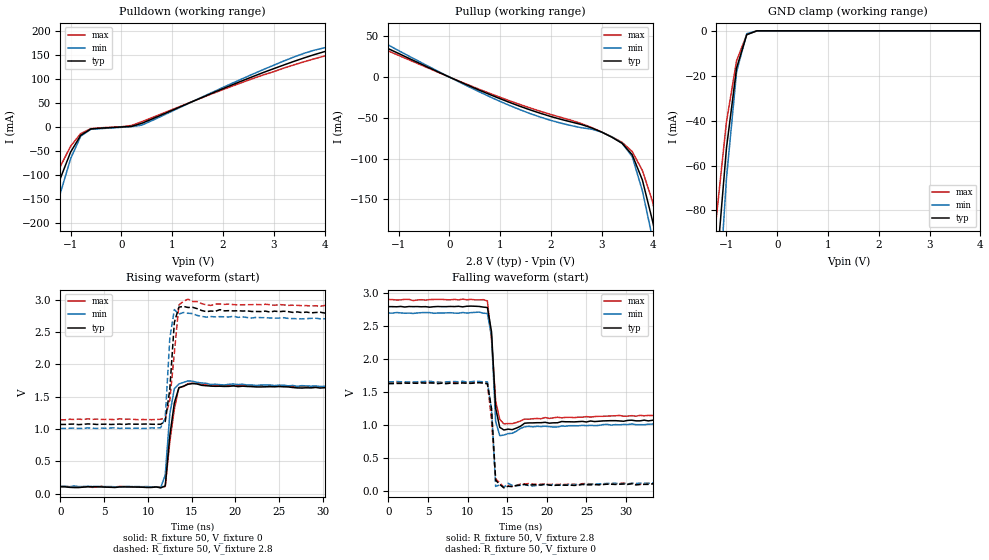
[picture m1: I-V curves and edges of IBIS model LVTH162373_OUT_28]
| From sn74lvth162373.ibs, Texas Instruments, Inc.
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|  Model LVTH162373 OUTPUT_28
[Model]   LVTH162373_OUT_28
Model_type  3-state
Polarity   Non-Inverting
Enable   Active-Low
Vmeas = 1.5V
Cref = 50pF
Rref = 500
Vref = 0
| variable   typ   min   max
C_comp   9p   NA   NA
[Temperature Range]   25   -40   85
[Voltage range]   2.8   2.7   2.9
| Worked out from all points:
|   slope of the pulldown table from 0 to 0.42 V, typ, clamps not added: 49.6 ohm
|   slope of the pullup table from 0 to 0.42 V, typ, clamps not added: 36.4 ohm
|   GND clamp passes 1 mA (typ) near -0.52 V on its own axis
|   rising waveform, R_fixture 50, V_fixture 0: 20-80 % time 769ps typ, 605ps min, 868ps max; typ from 0.108 V to 1.64 V
|   falling waveform, R_fixture 50, V_fixture 2.8: 20-80 % time 499ps typ, 417ps min, 672ps max; typ from 2.8 V to 1.07 V
|   rising waveform, R_fixture 50, V_fixture 2.8: 20-80 % time 628ps typ, 428ps min, 745ps max; typ from 1.07 V to 2.8 V
|   falling waveform, R_fixture 50, V_fixture 0: 20-80 % time 506ps typ, 502ps min, 629ps max; typ from 1.63 V to 0.112 V
[Pullup]
|   25C:2.8V   -40C:2.7V   85C:2.9V
|   Voltage   I(typ)   I(min)   I(max)
-5V       89.31uA    76.41uA    120.8uA
-2.8V     68.31uA    64.31uA    69.67uA
-2.6V     44.8mA     63.77uA    69.13uA
-2.4V     43.62mA    47.58mA    68.66uA
-1.8V     51.99mA    58.85mA    67.35uA
-1.4V     40.46mA    45.33mA    66.47uA
-1.2V     34.75mA    39.24mA    31.92mA
3.4V      -81.13mA   -81mA      -79.95mA
3.8V      -126.1mA   -139.3mA   -114.4mA
4V        -176.3mA   -197.6mA   -152.4mA
4.2V      -233.1mA   -255.9mA   -210.4mA
10V       -1.878A    -1.947A    -1.891A
[Pulldown]
|   25C:2.8V   -40C:2.7V   85C:2.9V
|   Voltage   I(typ)   I(min)   I(max)
-5V       -1.702A    -1.962A    -1.474A
-1.6V     -271.4mA   -329.1mA   -221.2mA
-1.4V     -187.3mA   -233.1mA   -147.5mA
-1.2V     -106.5mA   -137mA     -81.67mA
-1V       -52.21mA   -66.01mA   -39.97mA
-800mV    -17.24mA   -19.15mA   -13.68mA
-600mV    -4.145mA   -4.858mA   -3.442mA
400mV     7.456mA    3.702mA    10.86mA
3.8V      150.4mA    159.6mA    141.7mA
4.8V      173.8mA    180.6mA    164.4mA
6.6V      197.4mA    208mA      185.8mA
10V       230.8mA    256.2mA    213.8mA
[GND Clamp]
|   25C:2.8V   -40C:2.7V   85C:2.9V
|   Voltage   I(typ)   I(min)   I(max)
-5V       -1.686A    -1.93A     -1.49A
-1.4V     -187.1mA   -231mA     -150.5mA
-1.2V     -106.9mA   -136.6mA   -83.49mA
-1V       -52.29mA   -65.87mA   -40.6mA
-800mV    -16.54mA   -18.25mA   -13.27mA
-600mV    -1.712mA   -1.24mA    -1.686mA
-400mV    -7.76uA    -3.295uA   -12.98uA
5V        24.55nA    164nA      156.6nA
[ramp]
| variable   typ   min   max
dV/dt_r   9.360E-01/4.920E-10  9.420E-01/4.360E-10  9.480E-01/5.970E-10
dV/dt_f   1.056E+00/4.290E-10  1.032E+00/3.690E-10  1.074E+00/4.930E-10
R_load = 50
[Rising Waveform]
R_fixture = 50
V_fixture = 0
V_fixture_min = 0
V_fixture_max = 0
C_fixture = 0
L_fixture = 0
|   25C:2.8V   -40C:2.7V   85C:2.9V
|   Time   V(typ)   V(min)   V(max)
0s        107.9mV    117.2mV    112.6mV
11.46ns   91.71mV    95.83mV    103.6mV
11.98ns   121.6mV    290.1mV    112.9mV
12.5ns    893.9mV    1.229V     799.7mV
13.02ns   1.403V     1.623V     1.307V
13.54ns   1.636V     1.696V     1.64V
14.58ns   1.691V     1.743V     1.702V
17.19ns   1.663V     1.688V     1.673V
27.08ns   1.635V     1.661V     1.652V
50ns      1.635V     1.658V     1.655V
[Falling Waveform]
R_fixture = 50
V_fixture = 2.8
V_fixture_min = 2.7
V_fixture_max = 2.9
C_fixture = 0
L_fixture = 0
|   25C:2.8V   -40C:2.7V   85C:2.9V
|   Time   V(typ)   V(min)   V(max)
0s        2.796V     2.698V     2.903V
12.5ns    2.783V     2.692V     2.882V
13.02ns   2.415V     2.351V     2.295V
13.54ns   1.257V     1.055V     1.363V
14.06ns   964.5mV    839.2mV    1.084V
14.58ns   924.5mV    847.2mV    1.018V
15.63ns   929.6mV    874.3mV    1.02V
17.71ns   1.032V     979.8mV    1.088V
29.17ns   1.062V     1.003V     1.145V
50ns      1.071V     1.012V     1.147V
[Rising Waveform]
R_fixture = 50
V_fixture = 2.8
V_fixture_min = 2.7
V_fixture_max = 2.9
C_fixture = 0
L_fixture = 0
|   25C:2.8V   -40C:2.8V   85C:2.9V
|   Time   V(typ)   V(min)   V(max)
0s        1.071V     1.01V      1.143V
11.46ns   1.074V     1.021V     1.151V
11.98ns   1.118V     1.167V     1.173V
12.5ns    1.61V      2.399V     1.446V
13.02ns   2.645V     2.845V     2.171V
13.54ns   2.882V     2.774V     2.916V
14.58ns   2.877V     2.788V     3.006V
17.19ns   2.822V     2.737V     2.909V
33.85ns   2.797V     2.683V     2.898V
50ns      2.796V     2.7V       2.891V
[Falling Waveform]
R_fixture = 50
V_fixture = 0
V_fixture_min = 0
V_fixture_max = 0
C_fixture = 0
L_fixture = 0
|   25C:2.8V   -40C:2.7V   85C:2.9V
|   Time   V(typ)   V(min)   V(max)
0s        1.628V     1.655V     1.644V
12.5ns    1.626V     1.655V     1.631V
13.02ns   1.247V     1.234V     1.075V
13.54ns   162.4mV    68.51mV    180.5mV
14.06ns   98.42mV    89.72mV    121.6mV
14.58ns   46.39mV    55.85mV    58.59mV
15.1ns    70.19mV    114.9mV    73.09mV
18.23ns   94mV       74.46mV    103.8mV
34.9ns    111.7mV    125.4mV    123.1mV
50ns      112mV      111.4mV    106.2mV
